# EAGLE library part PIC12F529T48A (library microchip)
14-Pin, 8-Bit Flash Microcontrollers Source: 41634A.pdf
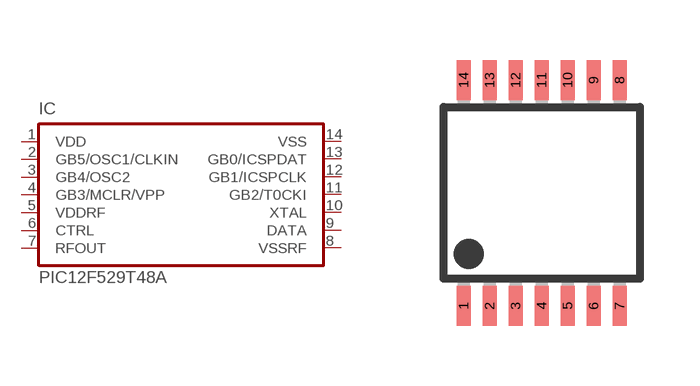
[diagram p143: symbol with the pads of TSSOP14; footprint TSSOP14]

Designator prefix IC

## PIC12F529T48A  [TSSOP14]
1  VDD  pwr
2  GB5/OSC1/CLKIN  hiz
3  GB4/OSC2  hiz
4  GB3/MCLR/VPP  in
5  VDDRF  in
6  CTRL  in
7  RFOUT  out
8  VSSRF  in
9  DATA  in
10  XTAL  in
11  GB2/T0CKI  hiz
12  GB1/ICSPCLK  hiz
13  GB0/ICSPDAT  hiz
14  VSS  pwr

## Footprint TSSOP14 (pad centres in mm)
14-Lead Plastic Thin Shrink Small Outline (ST) - 4.4 mm Body TSSOP Source: http://ww1.microchip.com/downloads/en/DeviceDoc/40039E.pdf
smd 0.35 x 1: 1 -1.95,-2.825; 2 -1.3,-2.825; 3 -0.65,-2.825; 4 0,-2.825; 5 0.65,-2.825; 6 1.3,-2.825; 7 1.95,-2.825; 8 1.95,2.825; 9 1.3,2.825; 10 0.65,2.825; 11 0,2.825; 12 -0.65,2.825; 13 -1.3,2.825; 14 -1.95,2.825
